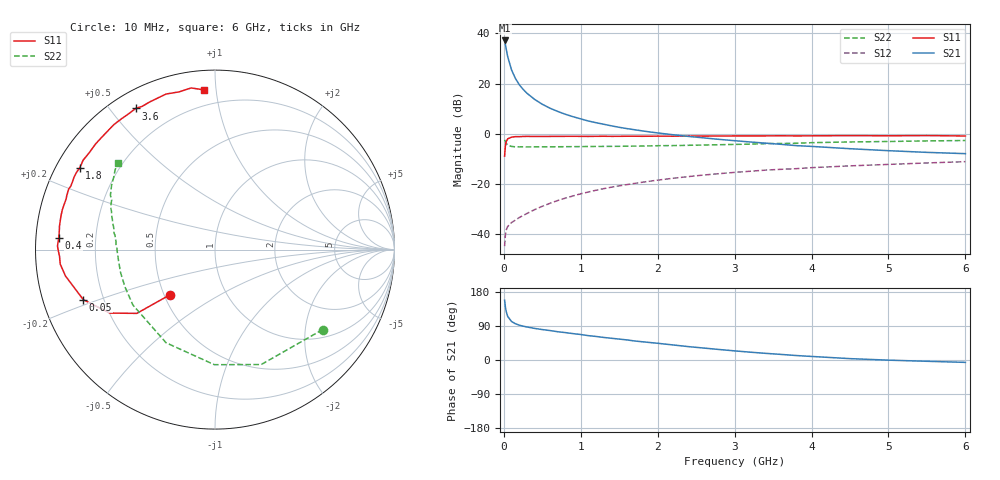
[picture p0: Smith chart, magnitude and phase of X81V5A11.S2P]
! SIEMENS Small Signal Semiconductors
! BFP136W
! Si NPN RF Bipolar Junction Transistor in SOT343
! VCE = 1.5 V  IC = 110 mA
! Common Emitter S-Parameters:  September  1994
# GHz  S  MA  R  50
!  f  S11  S21  S12  S22
! GHz  MAG  ANG  MAG  ANG  MAG  ANG  MAG  ANG
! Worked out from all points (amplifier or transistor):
!   40 points, 10 MHz to 6 GHz, reference 50 ohm
!   highest |S21| = 37.2 dB at 10 MHz (marker M1)
!   |S21| within 3 dB of that: start of sweep to 28.28 MHz
!   unconditionally stable (mu >= 1): 421 MHz to 3.225 GHz; 3.753 GHz to 3.865 GHz; 5.97 GHz to end of sweep
!   at 200 MHz: K = 0.75, MSG = 26.6 dB, |S12| = -33.6 dB
!   at 1.5 GHz: K = 1.12, MAG = 9.6 dB, |S12| = -20.9 dB
!   at 6 GHz: K = 1.00, MAG = 1.2 dB, |S12| = -11.2 dB
!   S11 on the Smith chart (normalised r, x): 10 MHz: 0.54, -0.31; 50 MHz: 0.12, -0.18; 400 MHz: 0.07, +0.04; 1.8 GHz: 0.07, +0.28; 3.6 GHz: 0.07, +0.58; 6 GHz: 0.11, +0.93
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0.01  0.3531 -134.8  72.53 157.9  0.0056 65.1  0.7473 -36.6
0.02  0.5624 -140.8  60.47 140.4  0.0093 55.6  0.6902 -68.1
0.03  0.6845 -148.9  49.63 128.5  0.0117 47.0  0.6413 -90.3
0.05  0.785 -159.2  34.5 115.0  0.0139 37.4  0.5863 -117.7
0.1  0.8461 -170.0  18.72 101.6  0.0166 36.7  0.5519 -146.0
0.15  0.8662 -174.7  12.67 95.7  0.0186 40.0  0.5428 -157.2
0.2  0.8668 -177.4  9.493 92.0  0.0209 43.9  0.5408 -163.1
0.25  0.8733 -179.7  7.66 89.3  0.023 46.7  0.5413 -166.8
0.3  0.8781 178.7  6.399 87.2  0.0252 50.1  0.5402 -169.4
0.4  0.8726 175.7  4.818 83.4  0.0301 54.2  0.541 -172.8
0.5  0.8738 173.1  3.843 80.3  0.0351 57.4  0.5418 -175.3
0.6  0.8763 171.3  3.209 77.7  0.0403 59.1  0.5427 -176.9
0.7  0.8775 168.9  2.767 74.6  0.0458 61.2  0.544 -178.1
0.9  0.8792 165.5  2.168 69.6  0.0565 62.1  0.5463 179.4
1.1  0.8762 161.2  1.777 64.2  0.0678 62.3  0.5501 177.8
1.8  0.8807 149.0  1.129 48.1  0.1063 58.8  0.5619 172.0
2.2  0.8845 142.3  0.944 39.7  0.1275 55.5  0.5736 168.8
3.2  0.8958 125.5  0.678 20.7  0.1761 45.4  0.6143 159.8
3.6  0.9021 119.3  0.609 14.8  0.1924 41.3  0.6328 156.2
4.5  0.9086 107.5  0.497 3.6  0.2255 32.6  0.6782 148.2
5.5  0.9103 98.4  0.42 -3.4  0.2579 24.7  0.7116 141.5
6  0.8926 94.1  0.396 -6.3  0.274 20.2  0.7245 138.5
